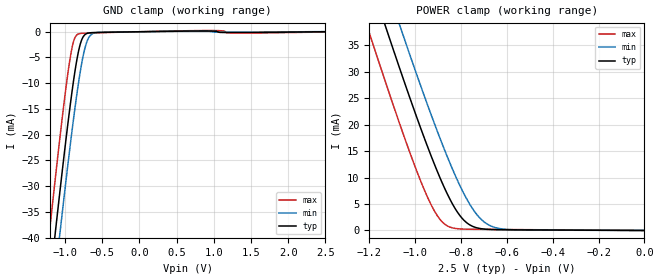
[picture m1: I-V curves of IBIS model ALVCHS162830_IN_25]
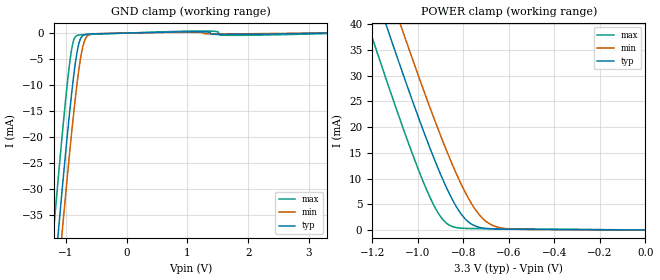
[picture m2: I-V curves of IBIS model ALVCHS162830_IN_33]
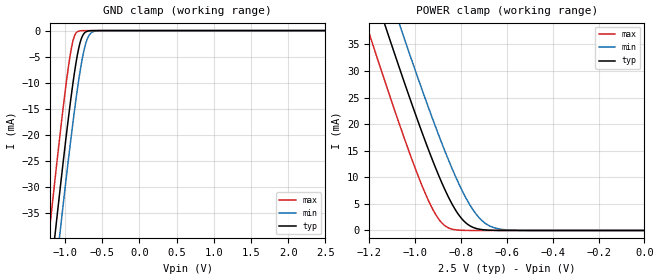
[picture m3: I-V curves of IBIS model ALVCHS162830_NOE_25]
| TEXAS INSTRUMENTS INCORPORATED
| Standard Linear and Logic Group
| IBIS Model of SN74ALVCHS162830
| 1-BIT TO 2-BIT ADDRESS DRIVER WITH 3-STATE OUTPUTS
| This file contains package information for the following:
|  TVSOP 80-pin (DBB) package as [Component] ALVCHS162830_DBB
| This device can be powered at the following Vccs:
|  2.5 volt Vcc
|  3.3 volt Vcc
| This file provides unique models under the [Model Selector] for each Vcc.
| For operation at a specific Vcc, select the appropriate model after each
| [Model Selector] keyword.
[IBIS Ver]   3.2
[Comment char]  |_char
[File Name]   sn74alvchs162830.ibs
[File Rev]   1.1 | no_rev
[Date]   November 3, 2000
[Source]   Data created from TI-SPICE simulations at TI-SLL.
[Notes]   The following is an IBIS list for the ALVCHS162830.
   Please contact sllibis@ti.com with questions and
   comments concerning SLL IBIS models.
   -Though we took all possible cautions, there are some
   Ramp End points mismatch warnings in this file.
   -Although all precautions were taken, there are still monotonic
   issues on various VI curves
[Disclaimer] Property of Texas Instruments Incorporated.  Unauthorized
   reproduction and/or distribution is strictly prohibited.
   This product is protected under copyright law.
   Created  2000, (C) Copyright  2000, Texas Instruments
   Incorporated, All Rights Reserved
   UNLESS THERE IS A SIGNED, WRITTEN AGREEMENT TO THE
   CONTRARY, TEXAS INSTRUMENTS (TI) IS PROVIDING THE IBIS
   MODELS  AND WITHOUT ANY WARRANTY, EXPRESSED OR
   IMPLIED.  TI assumes no liability for:
   1) the accuracy of the IBIS models provided to your
   company;
   2) the proper functioning of these IBIS Models in your
   design or for any resulting applications; or
   3) infringement of patents, copyrights or intellectual
   property rights resulting from your use of these IBIS
   models.
   TI provides IBIS Models as a service to our customers.
   You and your company shall not distribute, sell or give
   these models to anyone else without prior written
   permission from TI.
   TI reserves the right to make changes to our products or
   to discontinue any semiconductor product or service
   without notice, and advises our customers to obtain the
   latest version of relevant information to verify, before
   placing orders, that the information being relied on is
   current.
   Please be aware that your receipt and use of the IBIS
   information provided shall serve as acceptance of these
   terms and conditions.  If you do not accept these terms,
   you should return or destroy the IBIS models and any
   other accompanying information immediately.
| Component ALVCHS162830_DBB 80-pin TVSOP
[Component]   ALVCHS162830_DBB
[Manufacturer]   Texas Instruments, Inc.
[Package]
|   typ   min   max
R_pkg   8.300e-02   6.100e-02   1.190e-01
L_pkg   4.110e-09   3.114e-09   5.093e-09
C_pkg   5.670e-13   3.770e-13   7.860e-13
[Pin]   signal_name   model_name   R_pin   L_pin   C_pin
1   2Y2   ALVCHS162830_OUT   9.200e-02   4.977e-09   7.050e-13
2   1Y2   ALVCHS162830_OUT   8.900e-02   4.784e-09   7.860e-13
3   GND   GND   8.900e-02   4.801e-09   7.520e-13
4   2Y1   ALVCHS162830_OUT   9.600e-02   4.978e-09   7.780e-13
5   1Y1   ALVCHS162830_OUT   1.070e-01   5.093e-09   7.810e-13
6   VCC   POWER   1.120e-01   4.992e-09   7.250e-13
7   A1   ALVCHS162830_IN   1.150e-01   4.810e-09   6.690e-13
8   A2   ALVCHS162830_IN   1.190e-01   4.680e-09   6.140e-13
9   GND   GND   1.110e-01   4.446e-09   5.990e-13
10   A3   ALVCHS162830_IN   6.300e-02   4.077e-09   5.750e-13
11   A4   ALVCHS162830_IN   6.200e-02   3.905e-09   5.060e-13
12   GND   GND   6.500e-02   3.873e-09   4.920e-13
13   A5   ALVCHS162830_IN   6.500e-02   3.691e-09   4.730e-13
14   A6   ALVCHS162830_IN   6.500e-02   3.577e-09   4.590e-13
15   VCC   POWER   6.700e-02   3.487e-09   4.430e-13
16   A7   ALVCHS162830_IN   6.700e-02   3.343e-09   4.240e-13
17   A8   ALVCHS162830_IN   6.600e-02   3.262e-09   4.120e-13
18   GND   GND   6.800e-02   3.184e-09   3.950e-13
19   A9   ALVCHS162830_IN   6.900e-02   3.138e-09   3.770e-13
20   NOE1   ALVCHS162830_NOE   6.800e-02   3.114e-09   3.790e-13
21   NOE2   ALVCHS162830_NOE   6.800e-02   3.114e-09   3.790e-13
22   A10   ALVCHS162830_IN   6.900e-02   3.138e-09   3.770e-13
23   GND   GND   6.700e-02   3.184e-09   3.950e-13
24   A11   ALVCHS162830_IN   6.600e-02   3.262e-09   4.120e-13
25   A12   ALVCHS162830_IN   6.700e-02   3.343e-09   4.240e-13
26   VCC   POWER   6.700e-02   3.487e-09   4.430e-13
27   A13   ALVCHS162830_IN   6.500e-02   3.577e-09   4.590e-13
28   A14   ALVCHS162830_IN   6.500e-02   3.691e-09   4.730e-13
29   GND   GND   6.500e-02   3.873e-09   4.920e-13
30   A15   ALVCHS162830_IN   6.100e-02   3.902e-09   5.060e-13
31   A16   ALVCHS162830_IN   6.200e-02   4.073e-09   5.750e-13
32   GND   GND   1.110e-01   4.446e-09   5.990e-13
33   A17   ALVCHS162830_IN   1.190e-01   4.680e-09   6.140e-13
34   A18   ALVCHS162830_IN   1.140e-01   4.809e-09   6.690e-13
35   VCC   POWER   1.120e-01   4.993e-09   7.250e-13
36   2Y18   ALVCHS162830_OUT   1.070e-01   5.092e-09   7.810e-13
37   1Y18   ALVCHS162830_OUT   9.600e-02   4.979e-09   7.780e-13
38   GND   GND   8.900e-02   4.801e-09   7.520e-13
39   2Y17   ALVCHS162830_OUT   8.900e-02   4.783e-09   7.860e-13
40   1Y17   ALVCHS162830_OUT   9.200e-02   4.976e-09   7.050e-13
41   2Y16   ALVCHS162830_OUT   9.200e-02   4.975e-09   7.050e-13
42   1Y16   ALVCHS162830_OUT   8.900e-02   4.783e-09   7.860e-13
43   GND   GND   9.100e-02   4.807e-09   7.520e-13
44   2Y15   ALVCHS162830_OUT   9.600e-02   4.979e-09   7.780e-13
45   1Y15   ALVCHS162830_OUT   1.070e-01   5.092e-09   7.810e-13
46   VCC   POWER   1.120e-01   4.993e-09   7.250e-13
47   2Y14   ALVCHS162830_OUT   1.140e-01   4.809e-09   6.690e-13
48   1Y14   ALVCHS162830_OUT   1.190e-01   4.680e-09   6.140e-13
49   GND   GND   1.080e-01   4.439e-09   6.000e-13
50   2Y13   ALVCHS162830_OUT   6.200e-02   4.073e-09   5.760e-13
51   1Y13   ALVCHS162830_OUT   6.100e-02   3.903e-09   5.060e-13
52   GND   GND   6.500e-02   3.873e-09   4.920e-13
53   2Y12   ALVCHS162830_OUT   6.500e-02   3.691e-09   4.730e-13
54   1Y12   ALVCHS162830_OUT   6.600e-02   3.579e-09   4.590e-13
55   VCC   POWER   6.700e-02   3.487e-09   4.440e-13
56   2Y11   ALVCHS162830_OUT   6.700e-02   3.343e-09   4.250e-13
57   1Y11   ALVCHS162830_OUT   6.600e-02   3.262e-09   4.120e-13
58   GND   GND   6.800e-02   3.183e-09   3.950e-13
59   2Y10   ALVCHS162830_OUT   6.900e-02   3.139e-09   3.770e-13
60   1Y10   ALVCHS162830_OUT   6.800e-02   3.115e-09   3.790e-13
61   2Y9   ALVCHS162830_OUT   6.800e-02   3.115e-09   3.790e-13
62   1Y9   ALVCHS162830_OUT   6.900e-02   3.138e-09   3.770e-13
63   GND   GND   6.700e-02   3.183e-09   3.950e-13
64   2Y8   ALVCHS162830_OUT   6.600e-02   3.262e-09   4.120e-13
65   1Y8   ALVCHS162830_OUT   6.700e-02   3.343e-09   4.240e-13
66   VCC   POWER   6.700e-02   3.487e-09   4.440e-13
67   2Y7   ALVCHS162830_OUT   6.500e-02   3.577e-09   4.590e-13
68   1Y7   ALVCHS162830_OUT   6.500e-02   3.691e-09   4.730e-13
69   GND   GND   6.500e-02   3.873e-09   4.920e-13
70   2Y6   ALVCHS162830_OUT   6.200e-02   3.906e-09   5.060e-13
71   1Y6   ALVCHS162830_OUT   6.300e-02   4.077e-09   5.750e-13
72   GND   GND   1.080e-01   4.439e-09   6.000e-13
73   2Y5   ALVCHS162830_OUT   1.190e-01   4.679e-09   6.140e-13
74   1Y5   ALVCHS162830_OUT   1.150e-01   4.810e-09   6.690e-13
75   VCC   POWER   1.120e-01   4.993e-09   7.250e-13
76   2Y4   ALVCHS162830_OUT   1.070e-01   5.093e-09   7.800e-13
77   1Y4   ALVCHS162830_OUT   9.600e-02   4.978e-09   7.770e-13
78   GND   GND   9.100e-02   4.807e-09   7.520e-13
79   2Y3   ALVCHS162830_OUT   8.900e-02   4.784e-09   7.860e-13
80   1Y3   ALVCHS162830_OUT   9.200e-02   4.976e-09   7.050e-13
| Model ALVCHS162830_IN
[Model Selector]   ALVCHS162830_IN
ALVCHS162830_IN_25   2.5 volt Vcc
ALVCHS162830_IN_33   3.3 volt Vcc
| Model ALVCHS162830_NOE
[Model Selector]   ALVCHS162830_NOE
ALVCHS162830_NOE_25   2.5 volt Vcc
ALVCHS162830_NOE_33   3.3 volt Vcc
| Model ALVCHS162830_OUT
[Model Selector]   ALVCHS162830_OUT
ALVCHS162830_OUT_25   2.5 volt Vcc
ALVCHS162830_OUT_33   3.3 volt Vcc
| Models and submodels in the file (6): ALVCHS162830_IN_25 (Input), ALVCHS162830_IN_33 (Input), ALVCHS162830_NOE_25 (Input), ALVCHS162830_NOE_33 (Input), ALVCHS162830_OUT_25 (3-state), ALVCHS162830_OUT_33 (3-state)
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[Model]   ALVCHS162830_IN_25
Model_type  Input
Vinl = 0.7
Vinh = 1.7
| variable   typ   min   max
C_comp   6.15pF   5.70pF   6.73pF
[Temperature Range]   40   100   -40
| Ambient temperature   25   85   -40
[Voltage range]   2.5   2.3   2.7
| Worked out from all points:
|   GND clamp passes 1 mA (typ) near -0.76 V on its own axis
|   POWER clamp passes 1 mA (typ) near -0.76 V on its own axis
[GND Clamp]
| ALVCHS162830_IN_25
|   Voltage   I(typ)   I(min)   I(max)
-2.5V     -228.9mA   -236.3mA   -219.5mA
-1.23V    -51.94mA   -60.12mA   -41.46mA
-1.2V     -47.94mA   -56.13mA   -37.45mA
-1.13V    -38.73mA   -46.93mA   -28.23mA
-1.07V    -31.01mA   -39.17mA   -20.55mA
-925mV    -13.55mA   -21.28mA   -4.48mA
-880mV    -8.845mA   -16.16mA   -1.602mA
-830mV    -4.504mA   -10.9mA    -489.1uA
-775mV    -1.497mA   -5.972mA   -307.8uA
-720mV    -432uA     -2.485mA   -272.3uA
-610mV    -162.5uA   -253.6uA   -226.4uA
2.5V      6.607pA    26.34uA    -53.63uA
[POWER Clamp]
| ALVCHS162830_IN_25
|   Voltage   I(typ)   I(min)   I(max)
-2.5V     228.8mA    236.3mA    219.4mA
-1.22V    50.55mA    58.76mA    40.02mA
-1.185V   45.9mA     54.12mA    35.36mA
-1.125V   38.03mA    46.25mA    27.48mA
-1.07V    30.96mA    39.15mA    20.46mA
-1.055V   29.06mA    37.23mA    18.6mA
-960mV    17.47mA    25.42mA    7.672mA
-890mV    9.795mA    17.25mA    2.006mA
-795mV    2.296mA    7.611mA    274.9uA
-700mV    272.6uA    1.651mA    209.9uA
-590mV    125.7uA    168.7uA    174.5uA
-31.15fV  6.607pA    9.35pA     6.824pA
[Model]   ALVCHS162830_IN_33
Model_type  Input
Vinl = 0.8
Vinh = 2.0
| variable   typ   min   max
C_comp   6.02pF   5.58pF   7.06pF
[Temperature Range]   40   100   -40
| Ambient temperature   25   85   -40
[Voltage range]   3.3   3   3.6
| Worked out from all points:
|   GND clamp passes 1 mA (typ) near -0.76 V on its own axis
|   POWER clamp passes 1 mA (typ) near -0.76 V on its own axis
[GND Clamp]
| ALVCHS162830_IN_33
|   Voltage   I(typ)   I(min)   I(max)
-3.3V     -342.6mA   -349.7mA   -333.8mA
-1.215V   -50mA      -58.16mA   -39.53mA
-1.185V   -46.01mA   -54.19mA   -35.53mA
-1.125V   -38.14mA   -46.32mA   -27.65mA
-1.065V   -30.42mA   -38.57mA   -20mA
-925mV    -13.59mA   -21.32mA   -4.543mA
-875mV    -8.405mA   -15.64mA   -1.463mA
-820mV    -3.84mA    -9.958mA   -480.4uA
-770mV    -1.372mA   -5.616mA   -358uA
-715mV    -430.9uA   -2.286mA   -322uA
-585mV    -184.3uA   -197.4uA   -260.5uA
3.3V      8.596pA    50.87uA    -98.19uA
[POWER Clamp]
| ALVCHS162830_IN_33
|   Voltage   I(typ)   I(min)   I(max)
-3.3V     342.5mA    349.7mA    333.6mA
-1.24V    53.26mA    61.46mA    42.76mA
-1.2V     47.93mA    56.14mA    37.4mA
-1.125V   38.07mA    46.28mA    27.53mA
-1.065V   30.36mA    38.54mA    19.89mA
-960mV    17.51mA    25.45mA    7.717mA
-890mV    9.826mA    17.27mA    2.048mA
-795mV    2.326mA    7.633mA    313.8uA
-745mV    729.4uA    3.854mA    264.2uA
-700mV    299.5uA    1.67mA     245uA
-595mV    151.2uA    200.1uA    206.7uA
-48.03fV  8.596pA    11.09pA    9.035pA
[Model]   ALVCHS162830_NOE_25
Model_type  Input
Vinl = 0.7
Vinh = 1.7
| variable   typ   min   max
C_comp   6.66pF   6.14pF   7.15pF
[Temperature Range]   40   100   -40
| Ambient temperature   25   85   -40
[Voltage range]   2.5   2.3   2.7
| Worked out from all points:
|   GND clamp passes 1 mA (typ) near -0.77 V on its own axis
|   POWER clamp passes 1 mA (typ) near -0.77 V on its own axis
[GND Clamp]
| ALVCHS162830_NOE_25
|   Voltage   I(typ)   I(min)   I(max)
-2.5V     -228.1mA   -235.8mA   -218.5mA
-1.23V    -51.59mA   -59.87mA   -40.97mA
-1.2V     -47.61mA   -55.9mA    -36.97mA
-1.13V    -38.42mA   -46.71mA   -27.77mA
-1.07V    -30.71mA   -38.96mA   -20.13mA
-925mV    -13.29mA   -21.11mA   -4.122mA
-880mV    -8.606mA   -15.99mA   -1.263mA
-830mV    -4.281mA   -10.75mA   -171.6uA
-780mV    -1.472mA   -6.227mA   -17.15uA
-720mV    -242.5uA   -2.354mA   -1.023uA
-600mV    -3.832uA   -109.2uA   -3.611nA
2.5V      4.713pA    873.6pA    4.189pA
[POWER Clamp]
| ALVCHS162830_NOE_25
|   Voltage   I(typ)   I(min)   I(max)
-2.5V     228.1mA    235.8mA    218.5mA
-1.22V    50.26mA    58.55mA    39.63mA
-1.185V   45.62mA    53.91mA    34.98mA
-1.125V   37.77mA    46.06mA    27.13mA
-1.07V    30.71mA    38.96mA    20.13mA
-1.055V   28.82mA    37.05mA    18.27mA
-960mV    17.26mA    25.26mA    7.377mA
-890mV    9.597mA    17.1mA     1.734mA
-795mV    2.124mA    7.484mA    34.55uA
-700mV    123.8uA    1.543mA    399.1nA
-590mV    2.7uA      81.86uA    2.258nA
-31.15fV  4.713pA    6.963pA    4.886pA
